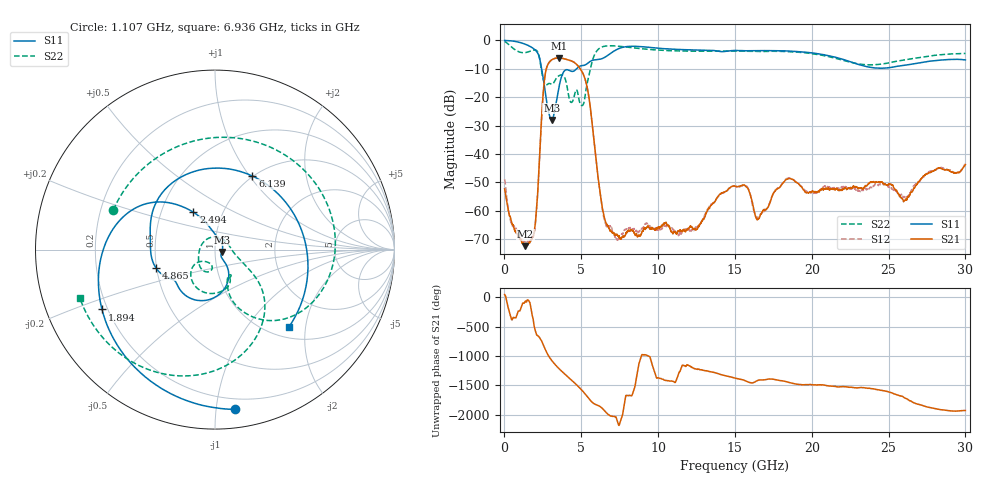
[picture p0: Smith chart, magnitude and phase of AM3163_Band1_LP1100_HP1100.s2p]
!Agilent Technologies,E8364B,MY43040894,A.07.50.67
!Agilent E8364B: A.07.50.67
!Date: Thursday, August 20, 2020 11:20:13
!Correction: S11(Full 2 Port(1,2))
!S21(Full 2 Port(1,2))
!S12(Full 2 Port(1,2))
!S22(Full 2 Port(1,2))
!S2P File: Measurements: S11, S21, S12, S22:
# Hz S  dB  R 50
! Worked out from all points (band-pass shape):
!   3201 points, 10 MHz to 30 GHz, reference 50 ohm
!   highest |S21| = -6.21 dB at 3.543 GHz (marker M1); lowest = -72.4 dB at 1.369 GHz (marker M2)
!   |S21| within 3 dB of the highest: 2.772 GHz to 4.815 GHz (2.044 GHz wide, 53.9 % of centre)
!   lowest |S11| = -28.0 dB at 3.075 GHz (marker M3), VSWR 1.08, Z = 53.9 - j1.45 ohm
!   |S11| at or under -10 dB: 2.418 GHz to 4.701 GHz (2.283 GHz wide, 64.1 % of centre)
!   |S22| runs from -23.0 to -0.4 dB; largest |S21 - S12| = 0.0052
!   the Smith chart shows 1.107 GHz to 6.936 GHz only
!   S11 on the Smith chart (normalised r, x): 1.107 GHz: 0.12, -1.13; 1.894 GHz: 0.18, -0.24; 2.494 GHz: 0.73, +0.32; 4.865 GHz: 0.50, -0.11; 6.139 GHz: 0.99, +1.03; 6.936 GHz: 1.22, -1.62
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1e7  -0.08 -5.0  -52.26 48.8  -48.82 19.3  -0.44 -15.5
4.5985e8  -0.24 -33.9  -63.88 -17.9  -64.60 -54.3  -2.39 -94.4
1.106509e9  -0.94 -82.7  -70.47 -158.9  -70.09 60.0  -4.32 158.7
1.368922e9  -1.43 -103.6  -72.39 -61.0  -71.15 -26.2  -4.33 118.3
1.893747e9  -2.95 -152.1  -68.95 -56.5  -68.67 -72.4  -3.46 31.7
2.493547e9  -12.40 120.0  -20.57 -67.2  -20.60 -67.2  -13.08 -71.5
3.074603e9  -28.04 -19.9  -6.91 5.0  -6.92 5.0  -15.46 -63.5
3.543197e9  -16.62 -59.0  -6.21 -133.4  -6.23 -133.3  -12.49 -83.0
4.096138e9  -10.36 -122.8  -6.82 92.6  -6.82 92.7  -17.00 -143.9
4.864631e9  -9.24 -163.1  -9.55 -94.9  -9.53 -95.0  -21.22 -177.9
5.014581e9  -8.94 -174.8  -10.75 -135.6  -10.73 -135.7  -22.93 100.3
6.139206e9  -6.75 63.0  -50.04 -50.1  -50.21 -51.7  -3.02 -98.3
6.935816e9  -4.50 -46.2  -67.19 136.4  -65.69 137.7  -1.94 -160.4
8.304109e9  -2.13 -169.3  -66.98 132.3  -66.51 121.5  -2.62 131.1
1.000979e10  -2.80 100.3  -65.70 66.9  -66.51 150.8  -3.48 63.4
1.224967e10  -3.41 10.7  -66.35 -121.1  -66.21 -114.1  -3.86 -14.3
1.5005e10  -3.61 -71.1  -51.35 63.9  -51.29 62.7  -3.82 -92.2
1.647638e10  -3.65 -107.1  -63.01 22.4  -62.36 10.4  -3.92 -128.4
2.000958e10  -4.44 163.4  -53.09 -49.7  -53.24 -51.1  -4.69 136.7
2.275554e10  -8.02 60.5  -51.44 -99.9  -52.10 -98.4  -8.02 21.3
2.500479e10  -9.67 -62.4  -50.66 -172.5  -51.60 -176.9  -7.98 -92.3
3e10  -6.91 104.9  -43.71 -129.0  -43.50 -126.1  -4.65 103.0
